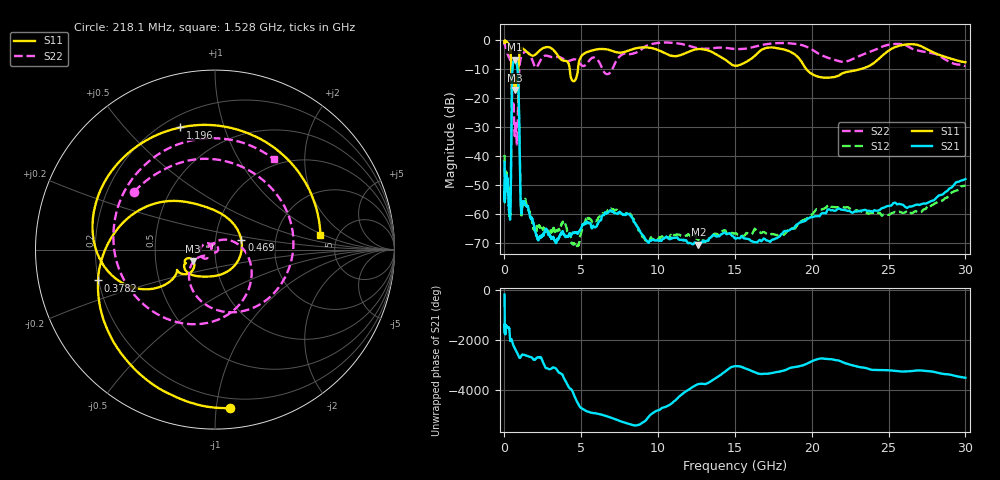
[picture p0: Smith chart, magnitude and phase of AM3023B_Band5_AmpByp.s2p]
# Hz S DB R 50.0
!freq dBS11 angS11 dBS21 angS21 dBS12 angS12 dBS22 angS22
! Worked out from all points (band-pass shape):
!   1601 points, 10 MHz to 30 GHz, reference 50 ohm
!   highest |S21| = -6.91 dB at 675.8 MHz (marker M1); lowest = -70.8 dB at 12.62 GHz (marker M2)
!   |S21| within 3 dB of the highest: 522.5 MHz to 846.5 MHz (324 MHz wide, 47.3 % of centre)
!   lowest |S11| = -17.3 dB at 699.9 MHz (marker M3), VSWR 1.32, Z = 38.9 - j5.01 ohm
!   |S11| at or under -10 dB: 443.1 MHz to 906.8 MHz (463.7 MHz wide, 68.7 % of centre); 4.245 GHz to 4.784 GHz (538.9 MHz wide, 11.9 % of centre); 19.63 GHz to 23.26 GHz (3.628 GHz wide, 16.9 % of centre)
!   |S22| runs from -36.2 to -0.9 dB; largest |S21 - S12| = 0.0097
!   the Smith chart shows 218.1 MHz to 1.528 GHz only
!   S11 on the Smith chart (normalised r, x): 218.1 MHz: 0.13, -1.09; 378.2 MHz: 0.20, -0.12; 469 MHz: 1.34, +0.15; 1.196 GHz: 0.26, +0.72; 1.528 GHz: 3.67, +0.90
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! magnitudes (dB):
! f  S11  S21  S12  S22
! 10 MHz  -0.4  -42.2  -39.7  -0.9
! 14.05 MHz  -1.1  -49.5  -51.5  -1.5
! 38.04 MHz  -0.2  -52.7  -51.7  -1.4
! 144.7 MHz  -0.6  -48.1  -47.7  -3.9
! 218.1 MHz  -1.0  -49.4  -49.1  -5.1
! 378.2 MHz  -3.4  -60.2  -59.7  -7.0
! 413.9 MHz  -5.4  -50.9  -52.0  -7.6
! 469 MHz  -16.1  -22.6  -22.5  -11.7
! 547.7 MHz  -14.4  -8.4  -8.4  -24.0
! 675.8 MHz  -16.7  -6.9  -6.9  -33.2
! 699.9 MHz  -17.3  -6.9  -6.9  -31.1
! 817.4 MHz  -12.4  -8.7  -8.7  -36.0
! 876.7 MHz  -11.8  -12.0  -12.0  -24.7
! 1.066 GHz  -2.9  -57.5  -57.8  -6.3
! 1.196 GHz  -3.0  -56.0  -56.9  -4.7
! 1.528 GHz  -4.5  -57.6  -58.5  -4.4
! 2.084 GHz  -4.8  -67.2  -65.3  -9.6
! 4.503 GHz  -14.3  -66.7  -70.3  -6.8
! 7.926 GHz  -4.0  -60.4  -59.9  -4.7
! 12.62 GHz  -3.2  -70.8  -69.1  -2.9
! 20.92 GHz  -13.1  -59.9  -58.0  -6.0
! 30 GHz  -7.7  -48.1  -50.3  -9.1
